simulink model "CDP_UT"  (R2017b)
settings: Solver=FixedStepDiscrete  StartTime=0.0  StopTime=10.0  FixedStep=0.01  RelTol=1e-3  EnableMultiTasking=on
undefined symbols (not defined in the file): ASWTYPE_FALSE, ASWTYPE_TRUE, CaCDP_CellTempNTCVoltTable_mV, CaCDP_CellTempTable_C, CaCDP_CMUPCBTempNTCVoltTable_mV, CaCDP_CMUPCBTempTable_C, CbCDP_DiffBusbarTempStateCheck_flg, CbCDP_DiffCellTempStateCheck_flg, CbCDP_DiffCellVoltStateCheck_flg, CbCDP_IgnorUpdateVld_flg, CbCDP_MaxBusbarTempStateCheck_flg, CbCDP_MaxCellTempStateCheck_flg, CbCDP_MaxCellVoltStateCheck_flg, CbCDP_MinBusbarTempStateCheck_flg, CbCDP_MinCellTempStateCheck_flg, CbCDP_MinCellVoltStateCheck_flg, CcCDP_AFETempConfig_numb, CcCDP_AFETempFltThd_C, CcCDP_AFETempFltThdHys_C, CcCDP_BusbarTempRngFltHiThrd_C, CcCDP_BusbarTempRngFltLowThrd_C, CcCDP_CellDiffFltLevel1_mV, CcCDP_CellDiffFltLevel2_mV, CcCDP_CellDiffFltLevel3_mV, CcCDP_CellTempLowerLimit_C, CcCDP_CellTempRngFltHiThrd_C, CcCDP_CellTempRngFltLowThrd_C, CcCDP_CellTempUpperLimit_C, CcCDP_CellVoltConfig_numb, CcCDP_CellVoltLowerLimit_mV, CcCDP_CellVoltRngHiThrd_mV, CcCDP_CellVoltRngLowThrd_mV, CcCDP_CellVoltUpdateThrd_numb, CcCDP_CellVoltUpperLimit_mV, CcCDP_ChrgMaxCellTempFltLv1Thrd_C, CcCDP_ChrgMaxCellTempFltLv2Thrd_C, CcCDP_ChrgMaxCellTempFltLv3Thrd_C, CcCDP_ChrgMaxCellTempReturnDiff_C, CcCDP_ChrgMinCellTempFltLv1Thrd_C, CcCDP_ChrgMinCellTempFltLv2Thrd_C, CcCDP_ChrgMinCellTempFltLv3Thrd_C, CcCDP_ChrgMinCellTempReturnDiff_C, CcCDP_CMUPCBTempConfig_numb, CcCDP_CMUPCBTempFltThd_C, CcCDP_CMUPCBTempFltThdHys_C, CcCDP_DiffBusbarTempFltLevel1Thrd_C, CcCDP_DiffBusbarTempFltLevel2Thrd_C, CcCDP_DiffBusbarTempReturnDifference_C, CcCDP_DiffCellTempFltLevel1Thrd_C, CcCDP_DiffCellTempFltLevel2Thrd_C, CcCDP_DiffCellTempReturnDifference_C, CcCDP_DiffCellVoltReturnDifference_mV, CcCDP_DiffVoltCheckMaxCellTempCondition_C, CcCDP_DiffVoltCheckMaxCellVoltCondition_mV, CcCDP_DiffVoltCheckMinCellTempCondition_C, CcCDP_DiffVoltCheckMinCellVoltCondition_mV, CcCDP_DiffVoltCheckPackCurrCondition_A, CcCDP_MaxAFETempIniVal_C, CcCDP_MaxBusbarTempFltLevel1Thrd_C, CcCDP_MaxBusbarTempFltLevel2Thrd_C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
libraries: AIWAYS_Powertrain_BMS_lib x148, simulink x8
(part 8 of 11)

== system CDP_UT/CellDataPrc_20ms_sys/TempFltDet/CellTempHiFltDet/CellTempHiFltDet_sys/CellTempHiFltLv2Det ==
  LbCDP_MaxTempCheckCondition_flg : Inport
  GcCDP_MaxCellTemp_C : Inport  Port=2
  Add1 : Sum  OutDataTypeStr=Inherit: Inherit via back propagation
  Add4 : Sum  OutDataTypeStr=Inherit: Inherit via back propagation
  CDP_GbCDP_ChrgMaxCellVoltFltLv1_flg : AIWAYS_Powertrain_BMS_lib/Signals/OverWrite  OverWrite_Value=CbCDP_CellTempHiFltLv2Ovr_flg  OverWrite_flag=CbCDP_CellTempHiFltLv2OvrSwt_flg
  Comparison : RelationalOperator  Operator=>  OutDataTypeStr=boolean
  Constant : Constant  Value=CcCDP_MaxCellTempFltLevel2Thrd_C
  Constant1 : Constant  Value=ASWTYPE_TRUE
  Constant2 : Constant  Value=CcCDP_MaxCellTempReturnDifference_C
  Constant3 : Constant  Value=CcCDP_MaxCellTempFltLevel3Thrd_C
  Constant4 : Constant  Value=CcCDP_MaxCellTempReturnDifference_C
  Constant5 : Constant  Value=ASWTYPE_TRUE
  Logical Operator : Logic  AllPortsSameDT=off  OutDataTypeStr=boolean
  Logical Operator1 : Logic  AllPortsSameDT=off  OutDataTypeStr=boolean
  Relational Operator : RelationalOperator  OutDataTypeStr=boolean
  Relational Operator1 : RelationalOperator  Operator===  OutDataTypeStr=boolean
  Terminator : Terminator
  GbCDP_CellTempHiFltLv2_flg : Outport
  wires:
  Constant2/1 -> Add4/2
  Logical Operator/1 -> CDP_GbCDP_ChrgMaxCellVoltFltLv1_flg/1
  Constant/1 -> Add4/1
  Add4/1 -> Relational Operator/2
  GcCDP_MaxCellTemp_C/1 -> Relational Operator/1, Comparison/2
  CDP_GbCDP_ChrgMaxCellVoltFltLv1_flg/1 -> GbCDP_CellTempHiFltLv2_flg/1  "GbCDP_CellTempHiFltLv2_flg"
  Relational Operator1/1 -> Logical Operator/2
  LbCDP_MaxTempCheckCondition_flg/1 -> Relational Operator1/1
  Constant1/1 -> Relational Operator1/2
  Relational Operator/1 -> Logical Operator1/2
  Constant4/1 -> Add1/2
  Constant3/1 -> Add1/1
  Add1/1 -> Comparison/1
  Comparison/1 -> Terminator/1
  Logical Operator1/1 -> Logical Operator/1
  Constant5/1 -> Logical Operator1/1

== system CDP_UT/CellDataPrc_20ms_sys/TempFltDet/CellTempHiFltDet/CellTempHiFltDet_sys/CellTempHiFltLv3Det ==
  LbCDP_MaxTempCheckCondition_flg : Inport
  GcCDP_MaxCellTemp_C : Inport  Port=2
  Add4 : Sum  OutDataTypeStr=Inherit: Inherit via back propagation
  CDP_GbCDP_ChrgMaxCellVoltFltLv1_flg : AIWAYS_Powertrain_BMS_lib/Signals/OverWrite  OverWrite_Value=CbCDP_CellTempHiFltLv3Ovr_flg  OverWrite_flag=CbCDP_CellTempHiFltLv3OvrSwt_flg
  Comparison : RelationalOperator  Operator=>  OutDataTypeStr=boolean
  Constant : Constant  Value=CcCDP_MaxCellTempFltLevel3Thrd_C
  Constant1 : Constant  Value=ASWTYPE_TRUE
  Constant2 : Constant  Value=CcCDP_MaxCellTempReturnDifference_C
  Constant3 : Constant  Value=CcCDP_CellTempRngFltHiThrd_C
  Constant4 : Constant  Value=ASWTYPE_TRUE
  Logical Operator : Logic  AllPortsSameDT=off  OutDataTypeStr=boolean
  Logical Operator1 : Logic  AllPortsSameDT=off  OutDataTypeStr=boolean
  Relational Operator : RelationalOperator  OutDataTypeStr=boolean
  Relational Operator1 : RelationalOperator  Operator===  OutDataTypeStr=boolean
  Terminator : Terminator
  GbCDP_CellTempHiFltLv3_flg : Outport
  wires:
  Logical Operator/1 -> CDP_GbCDP_ChrgMaxCellVoltFltLv1_flg/1
  CDP_GbCDP_ChrgMaxCellVoltFltLv1_flg/1 -> GbCDP_CellTempHiFltLv3_flg/1  "GbCDP_CellTempHiFltLv3_flg"
  Logical Operator1/1 -> Logical Operator/1
  Comparison/1 -> Terminator/1
  Relational Operator/1 -> Logical Operator1/2
  Constant/1 -> Add4/1
  Relational Operator1/1 -> Logical Operator/2
  Constant2/1 -> Add4/2
  Add4/1 -> Relational Operator/2
  LbCDP_MaxTempCheckCondition_flg/1 -> Relational Operator1/1
  Constant1/1 -> Relational Operator1/2
  GcCDP_MaxCellTemp_C/1 -> Relational Operator/1, Comparison/2
  Constant3/1 -> Comparison/1
  Constant4/1 -> Logical Operator1/1

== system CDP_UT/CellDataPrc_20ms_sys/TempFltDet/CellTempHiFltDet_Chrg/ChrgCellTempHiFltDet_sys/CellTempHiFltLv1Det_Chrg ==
  LbCDP_ChrgMaxTempChkCond_flg : Inport
  GcCDP_MaxCellTemp_C : Inport  Port=2
  Add1 : Sum  OutDataTypeStr=Inherit: Inherit via back propagation
  Add4 : Sum  OutDataTypeStr=Inherit: Inherit via back propagation
  CDP_GbCDP_ChrgMaxCellVoltFltLv1_flg : AIWAYS_Powertrain_BMS_lib/Signals/OverWrite  OverWrite_Value=CbCDP_ChrgCellTempHiFltLv1Ovr_flg  OverWrite_flag=CbCDP_ChrgCellTempHiFltLv1OvrSwt_flg
  Comparison : RelationalOperator  Operator=>  OutDataTypeStr=boolean
  Constant : Constant  Value=CcCDP_ChrgMaxCellTempFltLv1Thrd_C
  Constant1 : Constant  Value=ASWTYPE_TRUE
  Constant2 : Constant  Value=CcCDP_ChrgMaxCellTempReturnDiff_C
  Constant3 : Constant  Value=CcCDP_MaxCellTempFltLevel2Thrd_C
  Constant4 : Constant  Value=CcCDP_MaxCellTempReturnDifference_C
  Constant5 : Constant  Value=ASWTYPE_TRUE
  Logical Operator : Logic  AllPortsSameDT=off  OutDataTypeStr=boolean
  Logical Operator1 : Logic  AllPortsSameDT=off  OutDataTypeStr=boolean
  Relational Operator : RelationalOperator  OutDataTypeStr=boolean
  Relational Operator1 : RelationalOperator  Operator===  OutDataTypeStr=boolean
  Terminator : Terminator
  GbCDP_ChrgCellTempHiFltLv1_flg : Outport
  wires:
  Constant5/1 -> Logical Operator1/1
  GcCDP_MaxCellTemp_C/1 -> Comparison/2, Relational Operator/1
  Constant1/1 -> Relational Operator1/2
  LbCDP_ChrgMaxTempChkCond_flg/1 -> Relational Operator1/1
  Constant4/1 -> Add1/2
  Add4/1 -> Relational Operator/2
  Constant2/1 -> Add4/2
  Relational Operator1/1 -> Logical Operator/2
  Constant/1 -> Add4/1
  Relational Operator/1 -> Logical Operator1/2
  Constant3/1 -> Add1/1
  Comparison/1 -> Terminator/1
  Add1/1 -> Comparison/1
  Logical Operator1/1 -> Logical Operator/1
  CDP_GbCDP_ChrgMaxCellVoltFltLv1_flg/1 -> GbCDP_ChrgCellTempHiFltLv1_flg/1  "GbCDP_ChrgCellTempHiFltLv1_flg"
  Logical Operator/1 -> CDP_GbCDP_ChrgMaxCellVoltFltLv1_flg/1

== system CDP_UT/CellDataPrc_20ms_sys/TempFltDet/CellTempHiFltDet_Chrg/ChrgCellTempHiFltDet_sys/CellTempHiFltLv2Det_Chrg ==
  LbCDP_ChrgMaxTempChkCond_flg : Inport
  GcCDP_MaxCellTemp_C : Inport  Port=2
  Add1 : Sum  OutDataTypeStr=Inherit: Inherit via back propagation
  Add4 : Sum  OutDataTypeStr=Inherit: Inherit via back propagation
  CDP_GbCDP_ChrgMaxCellVoltFltLv1_flg : AIWAYS_Powertrain_BMS_lib/Signals/OverWrite  OverWrite_Value=CbCDP_ChrgCellTempHiFltLv2Ovr_flg  OverWrite_flag=CbCDP_ChrgCellTempHiFltLv2OvrSwt_flg
  Comparison : RelationalOperator  Operator=>  OutDataTypeStr=boolean
  Constant : Constant  Value=CcCDP_ChrgMaxCellTempFltLv2Thrd_C
  Constant1 : Constant  Value=ASWTYPE_TRUE
  Constant2 : Constant  Value=CcCDP_ChrgMaxCellTempReturnDiff_C
  Constant3 : Constant  Value=CcCDP_MaxCellTempFltLevel3Thrd_C
  Constant4 : Constant  Value=CcCDP_MaxCellTempReturnDifference_C
  Constant5 : Constant  Value=ASWTYPE_TRUE
  Logical Operator : Logic  AllPortsSameDT=off  OutDataTypeStr=boolean
  Logical Operator1 : Logic  AllPortsSameDT=off  OutDataTypeStr=boolean
  Relational Operator : RelationalOperator  OutDataTypeStr=boolean
  Relational Operator1 : RelationalOperator  Operator===  OutDataTypeStr=boolean
  Terminator : Terminator
  GbCDP_ChrgCellTempHiFltLv2_flg : Outport
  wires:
  Constant5/1 -> Logical Operator1/1
  Logical Operator1/1 -> Logical Operator/1
  Comparison/1 -> Terminator/1
  Add1/1 -> Comparison/1
  Constant3/1 -> Add1/1
  Constant4/1 -> Add1/2
  Relational Operator/1 -> Logical Operator1/2
  Constant1/1 -> Relational Operator1/2
  LbCDP_ChrgMaxTempChkCond_flg/1 -> Relational Operator1/1
  Relational Operator1/1 -> Logical Operator/2
  CDP_GbCDP_ChrgMaxCellVoltFltLv1_flg/1 -> GbCDP_ChrgCellTempHiFltLv2_flg/1  "GbCDP_ChrgCellTempHiFltLv2_flg"
  GcCDP_MaxCellTemp_C/1 -> Comparison/2, Relational Operator/1
  Add4/1 -> Relational Operator/2
  Constant/1 -> Add4/1
  Logical Operator/1 -> CDP_GbCDP_ChrgMaxCellVoltFltLv1_flg/1
  Constant2/1 -> Add4/2

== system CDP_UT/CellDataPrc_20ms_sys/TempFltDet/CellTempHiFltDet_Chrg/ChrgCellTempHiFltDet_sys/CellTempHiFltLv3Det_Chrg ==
  LbCDP_ChrgMaxTempChkCond_flg : Inport
  GcCDP_MaxCellTemp_C : Inport  Port=2
  Add4 : Sum  OutDataTypeStr=Inherit: Inherit via back propagation
  CDP_GbCDP_ChrgMaxCellVoltFltLv1_flg : AIWAYS_Powertrain_BMS_lib/Signals/OverWrite  OverWrite_Value=CbCDP_ChrgCellTempHiFltLv3Ovr_flg  OverWrite_flag=CbCDP_ChrgCellTempHiFltLv3OvrSwt_flg
  Comparison : RelationalOperator  Operator=>  OutDataTypeStr=boolean
  Constant : Constant  Value=CcCDP_ChrgMaxCellTempFltLv3Thrd_C
  Constant1 : Constant  Value=ASWTYPE_TRUE
  Constant2 : Constant  Value=CcCDP_ChrgMaxCellTempReturnDiff_C
  Constant3 : Constant  Value=CcCDP_CellTempRngFltHiThrd_C
  Constant4 : Constant  Value=ASWTYPE_TRUE
  Logical Operator : Logic  AllPortsSameDT=off  OutDataTypeStr=boolean
  Logical Operator1 : Logic  AllPortsSameDT=off  OutDataTypeStr=boolean
  Relational Operator : RelationalOperator  OutDataTypeStr=boolean
  Relational Operator1 : RelationalOperator  Operator===  OutDataTypeStr=boolean
  Terminator : Terminator
  GbCDP_ChrgCellTempHiFltLv3_flg : Outport
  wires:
  Constant4/1 -> Logical Operator1/1
  Constant3/1 -> Comparison/1
  GcCDP_MaxCellTemp_C/1 -> Comparison/2, Relational Operator/1
  Constant1/1 -> Relational Operator1/2
  LbCDP_ChrgMaxTempChkCond_flg/1 -> Relational Operator1/1
  Add4/1 -> Relational Operator/2
  Constant2/1 -> Add4/2
  Relational Operator1/1 -> Logical Operator/2
  Constant/1 -> Add4/1
  Relational Operator/1 -> Logical Operator1/2
  Comparison/1 -> Terminator/1
  Logical Operator1/1 -> Logical Operator/1
  CDP_GbCDP_ChrgMaxCellVoltFltLv1_flg/1 -> GbCDP_ChrgCellTempHiFltLv3_flg/1  "GbCDP_ChrgCellTempHiFltLv3_flg"
  Logical Operator/1 -> CDP_GbCDP_ChrgMaxCellVoltFltLv1_flg/1

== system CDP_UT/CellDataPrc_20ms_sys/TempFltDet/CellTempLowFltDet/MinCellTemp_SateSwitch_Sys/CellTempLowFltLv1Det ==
  GcCDP_MinCellTemp_C : Inport
  LbCDP_MinTempCheckCondition_flg : Inport  Port=2
  Add1 : Sum  Inputs=+-  OutDataTypeStr=Inherit: Inherit via back propagation
  Add4 : Sum  Inputs=+-  OutDataTypeStr=Inherit: Inherit via back propagation
  CDP_GbCDP_ChrgMaxCellVoltFltLv1_flg : AIWAYS_Powertrain_BMS_lib/Signals/OverWrite  OverWrite_Value=CbCDP_CellTempLowFltLv1Ovr_flg  OverWrite_flag=CbCDP_CellTempLowFltLv1OvrSwt_flg
  Comparison2 : RelationalOperator  Operator=<  OutDataTypeStr=boolean
  Constant : Constant  Value=CcCDP_MinCellTempFltLevel1Thrd_C
  Constant1 : Constant  Value=ASWTYPE_TRUE
  Constant2 : Constant  Value=CcCDP_MinCellTempReturnDifference_C
  Constant3 : Constant  Value=CcCDP_MinCellTempFltLevel2Thrd_C
  Constant4 : Constant  Value=CcCDP_MinCellTempReturnDifference_C
  Constant5 : Constant  Value=ASWTYPE_TRUE
  Logical Operator : Logic  AllPortsSameDT=off  OutDataTypeStr=boolean
  Logical Operator1 : Logic  AllPortsSameDT=off  OutDataTypeStr=boolean
  Relational Operator : RelationalOperator  Operator=<=  OutDataTypeStr=boolean
  Relational Operator1 : RelationalOperator  Operator===  OutDataTypeStr=boolean
  Terminator : Terminator
  GbCDP_CellTempLowFltLv1_flg : Outport
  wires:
  Logical Operator/1 -> CDP_GbCDP_ChrgMaxCellVoltFltLv1_flg/1
  CDP_GbCDP_ChrgMaxCellVoltFltLv1_flg/1 -> GbCDP_CellTempLowFltLv1_flg/1  "GbCDP_CellTempLowFltLv1_flg"
  Constant1/1 -> Relational Operator1/2
  LbCDP_MinTempCheckCondition_flg/1 -> Relational Operator1/1
  Constant2/1 -> Add4/2
  Add4/1 -> Relational Operator/2
  Relational Operator1/1 -> Logical Operator/2
  Add1/1 -> Comparison2/1
  Comparison2/1 -> Terminator/1
  Logical Operator1/1 -> Logical Operator/1
  Relational Operator/1 -> Logical Operator1/2
  Constant/1 -> Add4/1
  Constant4/1 -> Add1/2
  GcCDP_MinCellTemp_C/1 -> Relational Operator/1, Comparison2/2
  Constant3/1 -> Add1/1
  Constant5/1 -> Logical Operator1/1

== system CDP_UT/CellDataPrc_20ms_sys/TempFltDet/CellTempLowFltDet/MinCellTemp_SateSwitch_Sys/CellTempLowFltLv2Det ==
  GcCDP_MinCellTemp_C : Inport
  LbCDP_MinTempCheckCondition_flg : Inport  Port=2
  Add1 : Sum  Inputs=+-  OutDataTypeStr=Inherit: Inherit via back propagation
  Add4 : Sum  Inputs=+-  OutDataTypeStr=Inherit: Inherit via back propagation
  CDP_GbCDP_ChrgMaxCellVoltFltLv1_flg : AIWAYS_Powertrain_BMS_lib/Signals/OverWrite  OverWrite_Value=CbCDP_CellTempLowFltLv2Ovr_flg  OverWrite_flag=CbCDP_CellTempLowFltLv2OvrSwt_flg
  Comparison2 : RelationalOperator  Operator=<  OutDataTypeStr=boolean
  Constant : Constant  Value=CcCDP_MinCellTempFltLevel2Thrd_C
  Constant1 : Constant  Value=ASWTYPE_TRUE
  Constant2 : Constant  Value=CcCDP_MinCellTempReturnDifference_C
  Constant3 : Constant  Value=CcCDP_MinCellTempFltLevel3Thrd_C
  Constant4 : Constant  Value=CcCDP_MinCellTempReturnDifference_C
  Constant5 : Constant  Value=ASWTYPE_TRUE
  Logical Operator : Logic  AllPortsSameDT=off  OutDataTypeStr=boolean
  Logical Operator1 : Logic  AllPortsSameDT=off  OutDataTypeStr=boolean
  Relational Operator : RelationalOperator  Operator=<=  OutDataTypeStr=boolean
  Relational Operator1 : RelationalOperator  Operator===  OutDataTypeStr=boolean
  Terminator : Terminator
  GbCDP_CellTempLowFltLv2_flg : Outport
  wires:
  Constant/1 -> Add4/1
  GcCDP_MinCellTemp_C/1 -> Relational Operator/1, Comparison2/2
  Constant2/1 -> Add4/2
  Add4/1 -> Relational Operator/2
  Logical Operator/1 -> CDP_GbCDP_ChrgMaxCellVoltFltLv1_flg/1
  LbCDP_MinTempCheckCondition_flg/1 -> Relational Operator1/1
  Relational Operator1/1 -> Logical Operator/2
  Constant1/1 -> Relational Operator1/2
  CDP_GbCDP_ChrgMaxCellVoltFltLv1_flg/1 -> GbCDP_CellTempLowFltLv2_flg/1  "GbCDP_CellTempLowFltLv2_flg"
  Relational Operator/1 -> Logical Operator1/2
  Constant4/1 -> Add1/2
  Constant3/1 -> Add1/1
  Add1/1 -> Comparison2/1
  Comparison2/1 -> Terminator/1
  Logical Operator1/1 -> Logical Operator/1
  Constant5/1 -> Logical Operator1/1

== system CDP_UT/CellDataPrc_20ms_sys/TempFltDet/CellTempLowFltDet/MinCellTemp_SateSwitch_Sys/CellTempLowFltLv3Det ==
  GcCDP_MinCellTemp_C : Inport
  LbCDP_MinTempCheckCondition_flg : Inport  Port=2
  Add4 : Sum  Inputs=+-  OutDataTypeStr=Inherit: Inherit via back propagation
  CDP_GbCDP_ChrgMaxCellVoltFltLv1_flg : AIWAYS_Powertrain_BMS_lib/Signals/OverWrite  OverWrite_Value=CbCDP_CellTempLowFltLv3Ovr_flg  OverWrite_flag=CbCDP_CellTempLowFltLv3OvrSwt_flg
  Comparison2 : RelationalOperator  Operator=<  OutDataTypeStr=boolean
  Constant : Constant  Value=CcCDP_MinCellTempFltLevel3Thrd_C
  Constant1 : Constant  Value=ASWTYPE_TRUE
  Constant2 : Constant  Value=CcCDP_MinCellTempReturnDifference_C
  Constant3 : Constant  Value=CcCDP_CellTempRngFltHiThrd_C
  Constant4 : Constant  Value=ASWTYPE_TRUE
  Logical Operator : Logic  AllPortsSameDT=off  OutDataTypeStr=boolean
  Logical Operator1 : Logic  AllPortsSameDT=off  OutDataTypeStr=boolean
  Relational Operator : RelationalOperator  Operator=<=  OutDataTypeStr=boolean
  Relational Operator1 : RelationalOperator  Operator===  OutDataTypeStr=boolean
  Terminator : Terminator
  GbCDP_CellTempLowFltLv3_flg : Outport
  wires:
  Logical Operator/1 -> CDP_GbCDP_ChrgMaxCellVoltFltLv1_flg/1
  CDP_GbCDP_ChrgMaxCellVoltFltLv1_flg/1 -> GbCDP_CellTempLowFltLv3_flg/1  "GbCDP_CellTempLowFltLv3_flg"
  Constant1/1 -> Relational Operator1/2
  LbCDP_MinTempCheckCondition_flg/1 -> Relational Operator1/1
  Constant2/1 -> Add4/2
  Add4/1 -> Relational Operator/2
  Relational Operator1/1 -> Logical Operator/2
  Comparison2/1 -> Terminator/1
  Logical Operator1/1 -> Logical Operator/1
  Relational Operator/1 -> Logical Operator1/2
  Constant/1 -> Add4/1
  GcCDP_MinCellTemp_C/1 -> Comparison2/2, Relational Operator/1
  Constant3/1 -> Comparison2/1
  Constant4/1 -> Logical Operator1/1

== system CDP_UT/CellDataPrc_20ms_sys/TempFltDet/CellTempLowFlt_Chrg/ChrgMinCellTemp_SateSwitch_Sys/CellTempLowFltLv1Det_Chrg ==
  GcCDP_MinCellTemp_C : Inport
  LbCDP_ChrgMinTempChkCond_flg : Inport  Port=2
  Add1 : Sum  Inputs=+-  OutDataTypeStr=Inherit: Inherit via back propagation
  Add4 : Sum  Inputs=+-  OutDataTypeStr=Inherit: Inherit via back propagation
  CDP_GbCDP_ChrgMaxCellVoltFltLv1_flg : AIWAYS_Powertrain_BMS_lib/Signals/OverWrite  OverWrite_Value=CbCDP_ChrgCellTempLowFltLv1Ovr_flg  OverWrite_flag=CbCDP_ChrgCellTempLowFltLv1OvrSwt_flg
  Comparison2 : RelationalOperator  Operator=<  OutDataTypeStr=boolean
  Constant : Constant  Value=CcCDP_ChrgMinCellTempFltLv1Thrd_C
  Constant1 : Constant  Value=ASWTYPE_TRUE
  Constant2 : Constant  Value=CcCDP_ChrgMinCellTempReturnDiff_C
  Constant3 : Constant  Value=CcCDP_MinCellTempFltLevel2Thrd_C
  Constant4 : Constant  Value=CcCDP_MinCellTempReturnDifference_C
  Constant5 : Constant  Value=ASWTYPE_TRUE
  Logical Operator : Logic  AllPortsSameDT=off  OutDataTypeStr=boolean
  Logical Operator1 : Logic  AllPortsSameDT=off  OutDataTypeStr=boolean
  Relational Operator : RelationalOperator  Operator=<=  OutDataTypeStr=boolean
  Relational Operator1 : RelationalOperator  Operator===  OutDataTypeStr=boolean
  Terminator : Terminator
  GbCDP_ChrgCellTempLowFltLv1_flg : Outport
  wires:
  Constant5/1 -> Logical Operator1/1
  Constant3/1 -> Add1/1
  GcCDP_MinCellTemp_C/1 -> Comparison2/2, Relational Operator/1
  Constant4/1 -> Add1/2
  Constant/1 -> Add4/1
  Relational Operator/1 -> Logical Operator1/2
  Logical Operator1/1 -> Logical Operator/1
  Comparison2/1 -> Terminator/1
  Add1/1 -> Comparison2/1
  Relational Operator1/1 -> Logical Operator/2
  Add4/1 -> Relational Operator/2
  Constant2/1 -> Add4/2
  LbCDP_ChrgMinTempChkCond_flg/1 -> Relational Operator1/1
  Constant1/1 -> Relational Operator1/2
  CDP_GbCDP_ChrgMaxCellVoltFltLv1_flg/1 -> GbCDP_ChrgCellTempLowFltLv1_flg/1  "GbCDP_ChrgCellTempLowFltLv1_flg"
  Logical Operator/1 -> CDP_GbCDP_ChrgMaxCellVoltFltLv1_flg/1

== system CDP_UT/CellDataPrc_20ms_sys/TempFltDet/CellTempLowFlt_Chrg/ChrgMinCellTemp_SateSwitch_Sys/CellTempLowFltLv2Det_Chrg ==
  GcCDP_MinCellTemp_C : Inport
  LbCDP_ChrgMinTempChkCond_flg : Inport  Port=2
  Add1 : Sum  Inputs=+-  OutDataTypeStr=Inherit: Inherit via back propagation
  Add4 : Sum  Inputs=+-  OutDataTypeStr=Inherit: Inherit via back propagation
  CDP_GbCDP_ChrgMaxCellVoltFltLv1_flg : AIWAYS_Powertrain_BMS_lib/Signals/OverWrite  OverWrite_Value=CbCDP_ChrgCellTempLowFltLv2Ovr_flg  OverWrite_flag=CbCDP_ChrgCellTempLowFltLv2OvrSwt_flg
  Comparison2 : RelationalOperator  Operator=<  OutDataTypeStr=boolean
  Constant : Constant  Value=CcCDP_ChrgMinCellTempFltLv2Thrd_C
  Constant1 : Constant  Value=ASWTYPE_TRUE
  Constant2 : Constant  Value=CcCDP_ChrgMinCellTempReturnDiff_C
  Constant3 : Constant  Value=CcCDP_MinCellTempFltLevel3Thrd_C
  Constant4 : Constant  Value=CcCDP_MinCellTempReturnDifference_C
  Constant5 : Constant  Value=ASWTYPE_TRUE
  Logical Operator : Logic  AllPortsSameDT=off  OutDataTypeStr=boolean
  Logical Operator1 : Logic  AllPortsSameDT=off  OutDataTypeStr=boolean
  Relational Operator : RelationalOperator  Operator=<=  OutDataTypeStr=boolean
  Relational Operator1 : RelationalOperator  Operator===  OutDataTypeStr=boolean
  Terminator : Terminator
  GbCDP_ChrgCellTempLowFltLv2_flg : Outport
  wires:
  Constant5/1 -> Logical Operator1/1
  Logical Operator1/1 -> Logical Operator/1
  Comparison2/1 -> Terminator/1
  Add1/1 -> Comparison2/1
  Constant3/1 -> Add1/1
  Constant4/1 -> Add1/2
  Relational Operator/1 -> Logical Operator1/2
  CDP_GbCDP_ChrgMaxCellVoltFltLv1_flg/1 -> GbCDP_ChrgCellTempLowFltLv2_flg/1  "GbCDP_ChrgCellTempLowFltLv2_flg"
  Constant1/1 -> Relational Operator1/2
  Relational Operator1/1 -> Logical Operator/2
  LbCDP_ChrgMinTempChkCond_flg/1 -> Relational Operator1/1
  Logical Operator/1 -> CDP_GbCDP_ChrgMaxCellVoltFltLv1_flg/1
  Add4/1 -> Relational Operator/2
  Constant2/1 -> Add4/2
  GcCDP_MinCellTemp_C/1 -> Comparison2/2, Relational Operator/1
  Constant/1 -> Add4/1

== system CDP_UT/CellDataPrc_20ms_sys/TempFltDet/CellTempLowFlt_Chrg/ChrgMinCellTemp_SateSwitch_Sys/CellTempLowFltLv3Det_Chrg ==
  GcCDP_MinCellTemp_C : Inport
  LbCDP_ChrgMinTempChkCond_flg : Inport  Port=2
  Add4 : Sum  Inputs=+-  OutDataTypeStr=Inherit: Inherit via back propagation
  CDP_GbCDP_ChrgMaxCellVoltFltLv1_flg : AIWAYS_Powertrain_BMS_lib/Signals/OverWrite  OverWrite_Value=CbCDP_ChrgCellTempLowFltLv3Ovr_flg  OverWrite_flag=CbCDP_ChrgCellTempLowFltLv3OvrSwt_flg
  Comparison2 : RelationalOperator  Operator=<  OutDataTypeStr=boolean
  Constant : Constant  Value=CcCDP_ChrgMinCellTempFltLv3Thrd_C
  Constant1 : Constant  Value=ASWTYPE_TRUE
  Constant2 : Constant  Value=CcCDP_ChrgMinCellTempReturnDiff_C
  Constant3 : Constant  Value=CcCDP_CellTempRngFltHiThrd_C
  Constant4 : Constant  Value=ASWTYPE_TRUE
  Logical Operator : Logic  AllPortsSameDT=off  OutDataTypeStr=boolean
  Logical Operator1 : Logic  AllPortsSameDT=off  OutDataTypeStr=boolean
  Relational Operator : RelationalOperator  Operator=<=  OutDataTypeStr=boolean
  Relational Operator1 : RelationalOperator  Operator===  OutDataTypeStr=boolean
  Terminator : Terminator
  GbCDP_ChrgCellTempLowFltLv3_flg : Outport
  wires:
  Constant4/1 -> Logical Operator1/1
  Constant3/1 -> Comparison2/1
  GcCDP_MinCellTemp_C/1 -> Relational Operator/1, Comparison2/2
  Constant/1 -> Add4/1
  Relational Operator/1 -> Logical Operator1/2
  Logical Operator1/1 -> Logical Operator/1
  Comparison2/1 -> Terminator/1
  Relational Operator1/1 -> Logical Operator/2
  Add4/1 -> Relational Operator/2
  Constant2/1 -> Add4/2
  LbCDP_ChrgMinTempChkCond_flg/1 -> Relational Operator1/1
  Constant1/1 -> Relational Operator1/2
  CDP_GbCDP_ChrgMaxCellVoltFltLv1_flg/1 -> GbCDP_ChrgCellTempLowFltLv3_flg/1  "GbCDP_ChrgCellTempLowFltLv3_flg"
  Logical Operator/1 -> CDP_GbCDP_ChrgMaxCellVoltFltLv1_flg/1

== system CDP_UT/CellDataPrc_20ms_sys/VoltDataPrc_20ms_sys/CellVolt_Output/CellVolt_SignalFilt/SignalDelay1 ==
  u : Inport
  Bus to Vector : BusToVector
  Delay1Cycle : Subsystem
  Delay2Cycle : Subsystem
  Delay3Cycle : Subsystem
  Delay4Cycle : Subsystem
  Mux : Mux  Inputs=5
  y : Outport
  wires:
  u/1 -> Mux/1, Delay4Cycle/1(u), Delay3Cycle/1(u), Delay2Cycle/1(u), Delay1Cycle/1(u)
  Bus to Vector/1 -> y/1
  Delay4Cycle/1(y) -> Mux/5
  Delay2Cycle/1(y) -> Mux/3
  Delay3Cycle/1(y) -> Mux/4
  Delay1Cycle/1(y) -> Mux/2
  Mux/1 -> Bus to Vector/1

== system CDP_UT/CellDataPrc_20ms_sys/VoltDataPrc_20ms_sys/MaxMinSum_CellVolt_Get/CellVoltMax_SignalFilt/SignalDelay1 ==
  u : Inport
  Bus to Vector : BusToVector
  Delay1Cycle : Subsystem
  Delay2Cycle : Subsystem
  Delay3Cycle : Subsystem
  Delay4Cycle : Subsystem
  Mux : Mux  Inputs=5
  y : Outport
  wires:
  u/1 -> Mux/1, Delay4Cycle/1(u), Delay3Cycle/1(u), Delay2Cycle/1(u), Delay1Cycle/1(u)
  Bus to Vector/1 -> y/1
  Delay4Cycle/1(y) -> Mux/5
  Delay2Cycle/1(y) -> Mux/3
  Delay3Cycle/1(y) -> Mux/4
  Delay1Cycle/1(y) -> Mux/2
  Mux/1 -> Bus to Vector/1

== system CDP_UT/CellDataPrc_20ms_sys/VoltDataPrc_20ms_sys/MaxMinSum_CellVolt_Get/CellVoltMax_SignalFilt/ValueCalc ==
  Output_Value : Inport
  Output_index : Inport  Port=2
  CcCDP_CellVoltFilConfig_numb : Inport  Port=3
  Constant2 : Constant  Value=CDP_CONST1_NUMB
  Constant4 : Constant  Value=CDP_CONST2_NUMB
  Constant6 : Constant  Value=CDP_CONST1_NUMB
  Constant7 : Constant  Value=CDP_CONST2_NUMB
  Product1 : Product  Inputs=*/  OutDataTypeStr=Inherit: Inherit via back propagation
  Product2 : Product  Inputs=*/  OutDataTypeStr=Inherit: Inherit via back propagation
  Selector : Selector  InputPortWidth=5  IndexOptions=Index vector (port)  Indices=[1 3]  OutputSizes=1
  Selector1 : Selector  InputPortWidth=5  IndexOptions=Index vector (port)  Indices=[1 3]  OutputSizes=1
  Sum : Sum  OutDataTypeStr=Inherit: Inherit via back propagation  RndMeth=Zero
  Sum1 : Sum  OutDataTypeStr=Inherit: Inherit via back propagation  RndMeth=Zero
  GcCDP_MaxCellVolt_mV : Outport
  Output_index1 : Outport  Port=2
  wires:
  Selector1/1 -> Output_index1/1
  Selector/1 -> GcCDP_MaxCellVolt_mV/1
  Sum1/1 -> Product2/1
  Constant7/1 -> Product2/2
  Constant2/1 -> Sum/2
  Output_Value/1 -> Selector/1
  Constant6/1 -> Sum1/2
  Output_index/1 -> Selector1/1
  Sum/1 -> Product1/1
  Constant4/1 -> Product1/2
  Product1/1 -> Selector/2
  Product2/1 -> Selector1/2
  CcCDP_CellVoltFilConfig_numb/1 -> Sum/1, Sum1/1

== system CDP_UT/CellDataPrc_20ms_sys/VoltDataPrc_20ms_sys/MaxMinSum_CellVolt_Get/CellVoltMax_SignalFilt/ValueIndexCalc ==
  Output_index1 : Inport
  LcCDP_MaxCellVoltNumb_numb : Inport  Port=2
  LbCDP_CellVoltUpdateVld_flg : Inport  Port=3
  InputValueCalc1 : Stateflow chart  TreatAsAtomicUnit=on
  Selector2 : Selector  IndexMode=Zero-based  InputPortWidth=5  IndexOptions=Index vector (port)  Indices=[1 3]  OutputSizes=1
  Unit Delay1 : UnitDelay  SampleTime=-1  StateName=StateName
  GcCDP_MaxCellVoltNumb_numb : Outport
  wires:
  LbCDP_CellVoltUpdateVld_flg/1 -> InputValueCalc1/2(Rige)
  Output_index1/1 -> Selector2/2
  InputValueCalc1/1(Output_Value) -> Selector2/1, Unit Delay1/1
  Unit Delay1/1 -> InputValueCalc1/3(Old_Value)
  LcCDP_MaxCellVoltNumb_numb/1 -> InputValueCalc1/1(Input_Value)
  Selector2/1 -> GcCDP_MaxCellVoltNumb_numb/1

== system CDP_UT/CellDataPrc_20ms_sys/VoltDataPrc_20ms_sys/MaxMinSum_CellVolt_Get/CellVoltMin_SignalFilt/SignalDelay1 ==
  u : Inport
  Bus to Vector : BusToVector
  Delay1Cycle : Subsystem
  Delay2Cycle : Subsystem
  Delay3Cycle : Subsystem
  Delay4Cycle : Subsystem
  Mux : Mux  Inputs=5
  y : Outport
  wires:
  Mux/1 -> Bus to Vector/1
  Delay1Cycle/1(y) -> Mux/2
  Delay3Cycle/1(y) -> Mux/4
  Delay2Cycle/1(y) -> Mux/3
  Delay4Cycle/1(y) -> Mux/5
  Bus to Vector/1 -> y/1
  u/1 -> Delay1Cycle/1(u), Delay2Cycle/1(u), Delay3Cycle/1(u), Delay4Cycle/1(u), Mux/1

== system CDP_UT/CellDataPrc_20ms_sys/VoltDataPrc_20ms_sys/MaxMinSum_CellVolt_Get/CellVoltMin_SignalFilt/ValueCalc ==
  Output_Value : Inport
  Output_index : Inport  Port=2
  CcCDP_CellVoltFilConfig_numb : Inport  Port=3
  Constant2 : Constant  Value=CDP_CONST1_NUMB
  Constant4 : Constant  Value=CDP_CONST2_NUMB
  Constant6 : Constant  Value=CDP_CONST1_NUMB
  Constant7 : Constant  Value=CDP_CONST2_NUMB
  Product1 : Product  Inputs=*/  OutDataTypeStr=Inherit: Inherit via back propagation
  Product2 : Product  Inputs=*/  OutDataTypeStr=Inherit: Inherit via back propagation
  Selector : Selector  InputPortWidth=5  IndexOptions=Index vector (port)  Indices=[1 3]  OutputSizes=1
  Selector1 : Selector  InputPortWidth=5  IndexOptions=Index vector (port)  Indices=[1 3]  OutputSizes=1
  Sum : Sum  OutDataTypeStr=Inherit: Inherit via back propagation  RndMeth=Zero
  Sum1 : Sum  OutDataTypeStr=Inherit: Inherit via back propagation  RndMeth=Zero
  GcCDP_MinCellVolt_mV : Outport
  Output_index1 : Outport  Port=2
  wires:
  CcCDP_CellVoltFilConfig_numb/1 -> Sum1/1, Sum/1
  Product2/1 -> Selector1/2
  Product1/1 -> Selector/2
  Constant4/1 -> Product1/2
  Sum/1 -> Product1/1
  Output_index/1 -> Selector1/1
  Constant6/1 -> Sum1/2
  Output_Value/1 -> Selector/1
  Constant2/1 -> Sum/2
  Constant7/1 -> Product2/2
  Sum1/1 -> Product2/1
  Selector/1 -> GcCDP_MinCellVolt_mV/1
  Selector1/1 -> Output_index1/1

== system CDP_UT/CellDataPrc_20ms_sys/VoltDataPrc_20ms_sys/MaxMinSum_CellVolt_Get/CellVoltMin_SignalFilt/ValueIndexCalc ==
  Output_index1 : Inport
  LcCDP_MinCellVoltNumb_numb : Inport  Port=2
  LbCDP_CellVoltUpdateVld_flg : Inport  Port=3
  InputValueCalc1 : Stateflow chart  TreatAsAtomicUnit=on
  Selector2 : Selector  IndexMode=Zero-based  InputPortWidth=5  IndexOptions=Index vector (port)  Indices=[1 3]  OutputSizes=1
  Unit Delay1 : UnitDelay  SampleTime=-1  StateName=StateName
  GcCDP_MinCellVoltNumb_numb : Outport
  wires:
  LcCDP_MinCellVoltNumb_numb/1 -> InputValueCalc1/1(Input_Value)
  Unit Delay1/1 -> InputValueCalc1/3(Old_Value)
  InputValueCalc1/1(Output_Value) -> Unit Delay1/1, Selector2/1
  Output_index1/1 -> Selector2/2
  LbCDP_CellVoltUpdateVld_flg/1 -> InputValueCalc1/2(Rige)
  Selector2/1 -> GcCDP_MinCellVoltNumb_numb/1

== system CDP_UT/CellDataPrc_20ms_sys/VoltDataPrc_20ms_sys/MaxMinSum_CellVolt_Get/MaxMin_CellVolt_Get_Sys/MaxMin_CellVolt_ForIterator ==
  CcCDP_CellVoltConfig_numb : Inport
  LaCDP_CellVolt_mV : Inport  Port=2
  LaCDP_CellVoltVld_flg : Inport  Port=3
  Bus Creator : BusCreator  Inputs=3
  Bus Selector1 : BusSelector  OutputSignals=LcCDP_IniOutputCellVolt_mV,LcCDP_IniOutputCellVoltNumb_numb,LbCDP_IniOutputCellVoltVld_flg
  Bus Selector2 : BusSelector  OutputSignals=LcCDP_IniOutputCellVolt_mV,LcCDP_IniOutputCellVoltNumb_numb,LbCDP_IniOutputCellVoltVld_flg
  Data Type Conversion : DataTypeConversion
  MaxCellVoltNumbIterator : ForIterator  ResetStates=reset  IterationSource=external  IterationVariableDataType=int16
  MaxCellVoltNumb_ForIterator : Subsystem
  MinCellVoltNumb_ForIterator : Subsystem
  Selector : Selector  IndexOptions=Index vector (port)  Indices=[1 3]  OutputSizes=1
  Selector1 : Selector  IndexOptions=Index vector (port)  Indices=[1 3]  OutputSizes=1
  LcCDP_MaxCellVolt_mV : Outport
  LcCDP_MaxCellVoltNumb_numb : Outport  Port=2
  LcCDP_MinCellVolt_mV : Outport  Port=3
  LcCDP_MinCellVoltNumb_numb : Outport  Port=4
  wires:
  Bus Selector2/2 -> MinCellVoltNumb_ForIterator/2(LcCDP_IniOutputCellVoltNumb_numb)  "<LcCDP_IniOutputCellVoltNumb_numb>"
  Bus Selector2/1 -> MinCellVoltNumb_ForIterator/1(LcCDP_IniOutputCellVolt_mV)  "<LcCDP_IniOutputCellVolt_mV>"
  Bus Selector1/2 -> MaxCellVoltNumb_ForIterator/2(LcCDP_IniOutputCellVoltNumb_numb)  "<LcCDP_IniOutputCellVoltNumb_numb>"
  Bus Selector1/1 -> MaxCellVoltNumb_ForIterator/1(LcCDP_IniOutputCellVolt_mV)  "<LcCDP_IniOutputCellVolt_mV>"
  Data Type Conversion/1 -> Bus Creator/2  "LcCDP_IniOutputCellVoltNumb_numb"
  Bus Creator/1 -> Bus Selector2/1, Bus Selector1/1
  Selector/1 -> Bus Creator/1  "LcCDP_IniOutputCellVolt_mV"
  MaxCellVoltNumbIterator/1 -> Selector1/2, Data Type Conversion/1, Selector/2
  LaCDP_CellVolt_mV/1 -> Selector/1
  CcCDP_CellVoltConfig_numb/1 -> MaxCellVoltNumbIterator/1
  MaxCellVoltNumb_ForIterator/1(LcCDP_MaxCellVolt_mV) -> LcCDP_MaxCellVolt_mV/1
  MaxCellVoltNumb_ForIterator/2(LcCDP_MaxCellVoltNumb_numb) -> LcCDP_MaxCellVoltNumb_numb/1
  MinCellVoltNumb_ForIterator/1(LcCDP_MinCellVolt_mV) -> LcCDP_MinCellVolt_mV/1
  MinCellVoltNumb_ForIterator/2(LcCDP_MinCellVoltNumb_numb) -> LcCDP_MinCellVoltNumb_numb/1
  LaCDP_CellVoltVld_flg/1 -> Selector1/1
  Selector1/1 -> Bus Creator/3  "LbCDP_IniOutputCellVoltVld_flg"
  Bus Selector1/3 -> MaxCellVoltNumb_ForIterator/3(LbCDP_IniOutputCellVoltVld_flg)  "<LbCDP_IniOutputCellVoltVld_flg>"
  Bus Selector2/3 -> MinCellVoltNumb_ForIterator/3(LbCDP_IniOutputCellVoltVld_flg)  "<LbCDP_IniOutputCellVoltVld_flg>"

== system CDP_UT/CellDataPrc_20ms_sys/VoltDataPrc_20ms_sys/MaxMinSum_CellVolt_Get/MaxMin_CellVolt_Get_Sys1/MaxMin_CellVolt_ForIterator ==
  CcCDP_CellVoltConfig_numb : Inport
  LaCDP_CellVolt_mV : Inport  Port=2
  LaCDP_CellVoltVld_flg : Inport  Port=3
  Bus Creator : BusCreator  Inputs=3
  Bus Selector1 : BusSelector  OutputSignals=LcCDP_IniOutputCellVolt_mV,LcCDP_IniOutputCellVoltNumb_numb,LbCDP_IniOutputCellVoltVld_flg
  Bus Selector2 : BusSelector  OutputSignals=LcCDP_IniOutputCellVolt_mV,LcCDP_IniOutputCellVoltNumb_numb,LbCDP_IniOutputCellVoltVld_flg
  Data Type Conversion : DataTypeConversion
  MaxCellVoltNumbIterator : ForIterator  ResetStates=reset  IterationSource=external  IterationVariableDataType=int16
  MaxCellVoltNumb_ForIterator : Subsystem
  MinCellVoltNumb_ForIterator : Subsystem
  Selector : Selector  IndexOptions=Index vector (port)  Indices=[1 3]  OutputSizes=1
  Selector1 : Selector  IndexOptions=Index vector (port)  Indices=[1 3]  OutputSizes=1
  LcCDP_MaxCellVolt_mV : Outport
  LcCDP_MaxCellVoltNumb_numb : Outport  Port=2
  LcCDP_MinCellVolt_mV : Outport  Port=3
  LcCDP_MinCellVoltNumb_numb : Outport  Port=4
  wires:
  Bus Selector2/3 -> MinCellVoltNumb_ForIterator/3(LbCDP_IniOutputCellVoltVld_flg)  "<LbCDP_IniOutputCellVoltVld_flg>"
  Bus Selector1/3 -> MaxCellVoltNumb_ForIterator/3(LbCDP_IniOutputCellVoltVld_flg)  "<LbCDP_IniOutputCellVoltVld_flg>"
  Selector1/1 -> Bus Creator/3  "LbCDP_IniOutputCellVoltVld_flg"
  LaCDP_CellVoltVld_flg/1 -> Selector1/1
  MinCellVoltNumb_ForIterator/2(LcCDP_MinCellVoltNumb_numb) -> LcCDP_MinCellVoltNumb_numb/1
  MinCellVoltNumb_ForIterator/1(LcCDP_MinCellVolt_mV) -> LcCDP_MinCellVolt_mV/1
  MaxCellVoltNumb_ForIterator/2(LcCDP_MaxCellVoltNumb_numb) -> LcCDP_MaxCellVoltNumb_numb/1
  MaxCellVoltNumb_ForIterator/1(LcCDP_MaxCellVolt_mV) -> LcCDP_MaxCellVolt_mV/1
  CcCDP_CellVoltConfig_numb/1 -> MaxCellVoltNumbIterator/1
  LaCDP_CellVolt_mV/1 -> Selector/1
  MaxCellVoltNumbIterator/1 -> Selector/2, Data Type Conversion/1, Selector1/2
  Selector/1 -> Bus Creator/1  "LcCDP_IniOutputCellVolt_mV"
  Bus Creator/1 -> Bus Selector1/1, Bus Selector2/1
  Data Type Conversion/1 -> Bus Creator/2  "LcCDP_IniOutputCellVoltNumb_numb"
  Bus Selector1/1 -> MaxCellVoltNumb_ForIterator/1(LcCDP_IniOutputCellVolt_mV)  "<LcCDP_IniOutputCellVolt_mV>"
  Bus Selector1/2 -> MaxCellVoltNumb_ForIterator/2(LcCDP_IniOutputCellVoltNumb_numb)  "<LcCDP_IniOutputCellVoltNumb_numb>"
  Bus Selector2/1 -> MinCellVoltNumb_ForIterator/1(LcCDP_IniOutputCellVolt_mV)  "<LcCDP_IniOutputCellVolt_mV>"
  Bus Selector2/2 -> MinCellVoltNumb_ForIterator/2(LcCDP_IniOutputCellVoltNumb_numb)  "<LcCDP_IniOutputCellVoltNumb_numb>"

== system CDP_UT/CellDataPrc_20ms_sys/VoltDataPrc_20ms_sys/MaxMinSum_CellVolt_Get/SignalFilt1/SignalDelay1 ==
  u : Inport
  Bus to Vector : BusToVector
  Delay1Cycle : Subsystem
  Delay2Cycle : Subsystem
  Delay3Cycle : Subsystem
  Delay4Cycle : Subsystem
  Mux : Mux  Inputs=5
  y : Outport
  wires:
  Mux/1 -> Bus to Vector/1
  Delay1Cycle/1(y) -> Mux/2
  Delay3Cycle/1(y) -> Mux/4
  Delay2Cycle/1(y) -> Mux/3
  Delay4Cycle/1(y) -> Mux/5
  Bus to Vector/1 -> y/1
  u/1 -> Delay1Cycle/1(u), Delay2Cycle/1(u), Delay3Cycle/1(u), Delay4Cycle/1(u), Mux/1

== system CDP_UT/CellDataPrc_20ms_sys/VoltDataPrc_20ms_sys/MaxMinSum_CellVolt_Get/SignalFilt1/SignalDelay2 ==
  u : Inport
  Bus to Vector : BusToVector
  Delay1Cycle : Subsystem
  Delay2Cycle : Subsystem
  Delay3Cycle : Subsystem
  Delay4Cycle : Subsystem
  Mux : Mux  Inputs=5
  y : Outport
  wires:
  u/1 -> Mux/1, Delay4Cycle/1(u), Delay3Cycle/1(u), Delay2Cycle/1(u), Delay1Cycle/1(u)
  Bus to Vector/1 -> y/1
  Delay4Cycle/1(y) -> Mux/5
  Delay2Cycle/1(y) -> Mux/3
  Delay3Cycle/1(y) -> Mux/4
  Delay1Cycle/1(y) -> Mux/2
  Mux/1 -> Bus to Vector/1

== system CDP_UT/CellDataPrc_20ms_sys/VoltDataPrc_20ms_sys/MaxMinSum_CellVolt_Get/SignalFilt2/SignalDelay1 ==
  u : Inport
  Bus to Vector : BusToVector
  Delay1Cycle : Subsystem
  Delay2Cycle : Subsystem
  Delay3Cycle : Subsystem
  Delay4Cycle : Subsystem
  Mux : Mux  Inputs=5
  y : Outport
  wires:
  Mux/1 -> Bus to Vector/1
  Delay1Cycle/1(y) -> Mux/2
  Delay3Cycle/1(y) -> Mux/4
  Delay2Cycle/1(y) -> Mux/3
  Delay4Cycle/1(y) -> Mux/5
  Bus to Vector/1 -> y/1
  u/1 -> Delay1Cycle/1(u), Delay2Cycle/1(u), Delay3Cycle/1(u), Delay4Cycle/1(u), Mux/1

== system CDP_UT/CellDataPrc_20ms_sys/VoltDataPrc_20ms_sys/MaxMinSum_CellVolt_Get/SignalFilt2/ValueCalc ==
  Output_Value : Inport
  Output_index : Inport  Port=2
  CcCDP_CellVoltFilConfig_numb : Inport  Port=3
  Constant2 : Constant  Value=CDP_CONST1_NUMB
  Constant4 : Constant  Value=CDP_CONST2_NUMB
  Constant6 : Constant  Value=CDP_CONST1_NUMB
  Constant7 : Constant  Value=CDP_CONST2_NUMB
  Product1 : Product  Inputs=*/  OutDataTypeStr=Inherit: Inherit via back propagation
  Product2 : Product  Inputs=*/  OutDataTypeStr=Inherit: Inherit via back propagation
  Selector : Selector  InputPortWidth=5  IndexOptions=Index vector (port)  Indices=[1 3]  OutputSizes=1
  Selector1 : Selector  InputPortWidth=5  IndexOptions=Index vector (port)  Indices=[1 3]  OutputSizes=1
  Sum : Sum  OutDataTypeStr=Inherit: Inherit via back propagation  RndMeth=Zero
  Sum1 : Sum  OutDataTypeStr=Inherit: Inherit via back propagation  RndMeth=Zero
  Output_Value1 : Outport
  Output_index1 : Outport  Port=2
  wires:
  CcCDP_CellVoltFilConfig_numb/1 -> Sum1/1, Sum/1
  Product2/1 -> Selector1/2
  Product1/1 -> Selector/2
  Constant4/1 -> Product1/2
  Sum/1 -> Product1/1
  Output_index/1 -> Selector1/1
  Constant6/1 -> Sum1/2
  Output_Value/1 -> Selector/1
  Constant2/1 -> Sum/2
  Constant7/1 -> Product2/2
  Sum1/1 -> Product2/1
  Selector/1 -> Output_Value1/1
  Selector1/1 -> Output_index1/1

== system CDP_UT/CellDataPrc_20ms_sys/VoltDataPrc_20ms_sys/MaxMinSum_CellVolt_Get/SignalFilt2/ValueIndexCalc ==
  Output_index1 : Inport
  Input_Numb : Inport  Port=2
  InputValueVld : Inport  Port=3
  InputValueUpdate : Inport  Port=4
  Comparison4 : RelationalOperator  Operator===  OutDataTypeStr=boolean
  Constant1 : Constant  Value=CDP_CONST0_NUMB
  EdgeBi : AIWAYS_Powertrain_BMS_lib/Logical Operators/EdgeBi
  InputValueCalc1 : Stateflow chart  TreatAsAtomicUnit=on
  Logical : Logic  OutDataTypeStr=boolean
  Selector2 : Selector  IndexMode=Zero-based  InputPortWidth=5  IndexOptions=Index vector (port)  Indices=[1 3]  OutputSizes=1
  Unit Delay1 : UnitDelay  SampleTime=-1  StateName=StateName
  Output_Numb : Outport
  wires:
  Selector2/1 -> Output_Numb/1
  EdgeBi/1 -> InputValueCalc1/2(Rige)
  Input_Numb/1 -> InputValueCalc1/1(Input_Value)
  Unit Delay1/1 -> InputValueCalc1/3(Old_Value)
  InputValueCalc1/1(Output_Value) -> Unit Delay1/1, Selector2/1
  Output_index1/1 -> Selector2/2
  InputValueVld/1 -> Logical/1
  Constant1/1 -> Comparison4/2
  InputValueUpdate/1 -> Comparison4/1
  Comparison4/1 -> Logical/2
  Logical/1 -> EdgeBi/1

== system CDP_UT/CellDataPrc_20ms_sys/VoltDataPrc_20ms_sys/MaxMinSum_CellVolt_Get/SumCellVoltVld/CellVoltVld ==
  LaCDP_CellVoltVld_flg : Inport
  CcCDP_CellVoltConfig_numb : Inport  Port=2
  CellVolt : ForIterator  ResetStates=reset  IterationSource=external  IterationVariableDataType=int16
  Comparison1 : RelationalOperator  OutDataTypeStr=boolean
  Constant4 : Constant  Value=CcCDP_CellVoltUpdateThrd_numb
  Data Type Conversion : DataTypeConversion
  Logical Operator : Logic  Operator=OR  AllPortsSameDT=off  OutDataTypeStr=boolean
  Logical Operator1 : Logic  AllPortsSameDT=off  OutDataTypeStr=boolean
  Selector : Selector  IndexOptions=Index vector (port)  Indices=[1 3]  OutputSizes=1
  Sum : Sum  OutDataTypeStr=Inherit: Inherit via back propagation  RndMeth=Zero
  Unit Delay : UnitDelay  InitialCondition=ASWTYPE_TRUE  SampleTime=-1  StateName=StateName
  Unit Delay1 : UnitDelay  SampleTime=-1  StateName=StateName
  Unit Delay2 : UnitDelay  SampleTime=-1  StateName=StateName
  LbCDP_AnyCellVoltVld_flg : Outport
  LbCDP_SumCellVoltVld_flg : Outport  Port=2
  LbCDP_CellVoltUpdateVld_flg : Outport  Port=3
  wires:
  Selector/1 -> Logical Operator1/1, Logical Operator/1, Data Type Conversion/1
  CellVolt/1 -> Selector/2
  CcCDP_CellVoltConfig_numb/1 -> CellVolt/1
  Logical Operator/1 -> Unit Delay1/1, LbCDP_AnyCellVoltVld_flg/1  "LbCDP_AnyCellVoltVld_flg"
  LaCDP_CellVoltVld_flg/1 -> Selector/1
  Logical Operator1/1 -> Unit Delay/1, LbCDP_SumCellVoltVld_flg/1  "LbCDP_SumCellVoltVld_flg"
  Unit Delay/1 -> Logical Operator1/2
  Unit Delay1/1 -> Logical Operator/2
  Data Type Conversion/1 -> Sum/2
  Sum/1 -> Comparison1/1, Unit Delay2/1
  Unit Delay2/1 -> Sum/1
  Constant4/1 -> Comparison1/2
  Comparison1/1 -> LbCDP_CellVoltUpdateVld_flg/1  "LbCDP_CellVoltUpdateVld_flg"

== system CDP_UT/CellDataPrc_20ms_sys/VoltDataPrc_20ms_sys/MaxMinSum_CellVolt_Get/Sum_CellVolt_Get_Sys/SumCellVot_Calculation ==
  LcCDP_SumCellVolt_mV : Inport
  Constant : Constant  Value=CDP_MV2V_NUMB
  Constant1 : Constant  Value=CcCDP_CellVoltConfig_numb
  Data Type Conversion : DataTypeConversion
  Divide1 : Product  Inputs=*/  OutDataTypeStr=single
  Divide2 : Product  Inputs=/*  OutDataTypeStr=single
  OverWrite1 : AIWAYS_Powertrain_BMS_lib/Signals/OverWrite  OverWrite_Value=CcCDP_AvgCellVoltOvr_mV  OverWrite_flag=CbCDP_AvgCellVoltOvrSwt_flg
  OverWrite2 : AIWAYS_Powertrain_BMS_lib/Signals/OverWrite  OverWrite_Value=CcCDP_SumCellVoltOvr_V  OverWrite_flag=CbCDP_SumCellVoltOvrSwt_flg
  GcCDP_SumCellVolt_V : Outport
  GcCDP_AvgCellVolt_mV : Outport  Port=2
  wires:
  Divide2/1 -> OverWrite2/1
  Constant/1 -> Divide2/1
  OverWrite2/1 -> GcCDP_SumCellVolt_V/1  "GcCDP_SumCellVolt_V"
  LcCDP_SumCellVolt_mV/1 -> Divide1/1, Divide2/2
  Constant1/1 -> Divide1/2
  Divide1/1 -> Data Type Conversion/1
  Data Type Conversion/1 -> OverWrite1/1
  OverWrite1/1 -> GcCDP_AvgCellVolt_mV/1  "GcCDP_AvgCellVolt_mV"

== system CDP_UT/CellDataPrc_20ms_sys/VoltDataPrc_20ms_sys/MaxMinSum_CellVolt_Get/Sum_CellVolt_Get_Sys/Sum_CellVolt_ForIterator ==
  CcCDP_CellVoltConfig_numb : Inport
  LaCDP_CellVolt_mV : Inport  Port=2
  Add : Sum  OutDataTypeStr=Inherit: Inherit via back propagation
  MaxCellVoltNumbIterator : ForIterator  ResetStates=reset  IterationSource=external  IterationVariableDataType=int16
  Selector : Selector  IndexOptions=Index vector (port)  Indices=[1 3]  OutputSizes=1
  Unit Delay : UnitDelay  SampleTime=-1  StateName=StateName
  LcCDP_SumCellVolt_mV : Outport
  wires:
  Selector/1 -> Add/2  "LcCDP_IniOutputSumCellVolt_mV"
  MaxCellVoltNumbIterator/1 -> Selector/2
  LaCDP_CellVolt_mV/1 -> Selector/1
  CcCDP_CellVoltConfig_numb/1 -> MaxCellVoltNumbIterator/1
  Add/1 -> Unit Delay/1, LcCDP_SumCellVolt_mV/1  "LcCDP_SumCellVolt_mV"
  Unit Delay/1 -> Add/1

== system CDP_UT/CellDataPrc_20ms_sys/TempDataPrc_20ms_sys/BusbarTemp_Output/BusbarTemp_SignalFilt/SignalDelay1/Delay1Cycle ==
  u : Inport
  Constant2 : Constant  Value=ASWTYPE_FALSE
  Switch : Switch  Criteria=u2 ~= 0  Threshold=1  RndMeth=Zero
  Unit Delay1 : UnitDelay  SampleTime=-1  StateName=StateName
  Unit Delay21 : UnitDelay  InitialCondition=1  SampleTime=-1  StateName=StateName
  y : Outport
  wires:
  Switch/1 -> y/1
  u/1 -> Switch/1, Unit Delay1/1
  Unit Delay1/1 -> Switch/3
  Unit Delay21/1 -> Switch/2
  Constant2/1 -> Unit Delay21/1

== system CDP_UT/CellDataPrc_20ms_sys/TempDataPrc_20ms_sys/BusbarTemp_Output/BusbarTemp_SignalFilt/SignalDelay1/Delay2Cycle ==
  u : Inport
  Constant2 : Constant  Value=ASWTYPE_FALSE
  Switch : Switch  Criteria=u2 ~= 0  Threshold=1  RndMeth=Zero
  Unit Delay1 : UnitDelay  SampleTime=-1  StateName=StateName
  Unit Delay2 : UnitDelay  InitialCondition=1  SampleTime=-1  StateName=StateName
  Unit Delay21 : UnitDelay  InitialCondition=1  SampleTime=-1  StateName=StateName
  Unit Delay3 : UnitDelay  SampleTime=-1  StateName=StateName
  y : Outport
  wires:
  Unit Delay3/1 -> Switch/3
  Unit Delay2/1 -> Switch/2
  Constant2/1 -> Unit Delay21/1
  Unit Delay21/1 -> Unit Delay2/1
  Unit Delay1/1 -> Unit Delay3/1
  u/1 -> Unit Delay1/1, Switch/1
  Switch/1 -> y/1

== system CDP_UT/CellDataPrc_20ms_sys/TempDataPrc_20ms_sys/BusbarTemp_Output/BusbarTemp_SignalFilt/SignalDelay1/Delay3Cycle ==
  u : Inport
  Constant2 : Constant  Value=ASWTYPE_FALSE
  Switch : Switch  Criteria=u2 ~= 0  Threshold=1  RndMeth=Zero
  Unit Delay1 : UnitDelay  SampleTime=-1  StateName=StateName
  Unit Delay2 : UnitDelay  InitialCondition=1  SampleTime=-1  StateName=StateName
  Unit Delay21 : UnitDelay  InitialCondition=1  SampleTime=-1  StateName=StateName
  Unit Delay3 : UnitDelay  SampleTime=-1  StateName=StateName
  Unit Delay4 : UnitDelay  InitialCondition=1  SampleTime=-1  StateName=StateName
  Unit Delay5 : UnitDelay  SampleTime=-1  StateName=StateName
  y : Outport
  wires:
  Unit Delay5/1 -> Switch/3
  Unit Delay4/1 -> Switch/2
  Unit Delay3/1 -> Unit Delay5/1
  Unit Delay2/1 -> Unit Delay4/1
  Constant2/1 -> Unit Delay21/1
  Unit Delay21/1 -> Unit Delay2/1
  Unit Delay1/1 -> Unit Delay3/1
  u/1 -> Unit Delay1/1, Switch/1
  Switch/1 -> y/1

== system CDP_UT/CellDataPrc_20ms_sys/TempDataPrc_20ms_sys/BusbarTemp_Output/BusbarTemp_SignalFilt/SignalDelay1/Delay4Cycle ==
  u : Inport
  Constant2 : Constant  Value=ASWTYPE_FALSE
  Switch : Switch  Criteria=u2 ~= 0  Threshold=1  RndMeth=Zero
  Unit Delay{1,3,5,7} (4 alike) : UnitDelay  SampleTime=-1  StateName=StateName
  Unit Delay{2,4,6,21} (4 alike) : UnitDelay  InitialCondition=1  SampleTime=-1  StateName=StateName
  y : Outport
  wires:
  Unit Delay7/1 -> Switch/3
  Unit Delay6/1 -> Switch/2
  Unit Delay5/1 -> Unit Delay7/1
  Unit Delay4/1 -> Unit Delay6/1
  Unit Delay3/1 -> Unit Delay5/1
  Unit Delay2/1 -> Unit Delay4/1
  Constant2/1 -> Unit Delay21/1
  Unit Delay21/1 -> Unit Delay2/1
  Unit Delay1/1 -> Unit Delay3/1
  u/1 -> Unit Delay1/1, Switch/1
  Switch/1 -> y/1

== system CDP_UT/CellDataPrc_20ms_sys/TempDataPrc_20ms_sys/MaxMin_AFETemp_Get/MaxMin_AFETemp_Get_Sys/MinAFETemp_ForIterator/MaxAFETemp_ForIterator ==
  LcCDP_IniOutputAFETemp_C : Inport
  LcCDP_IniOutputAFETempNumb_numb : Inport  Port=2
  LbCDP_IniOutputAFETempVld_flg : Inport  Port=3
  Constant3 : Constant  Value=CcCDP_MaxAFETempIniVal_C
  Logical Operator : Logic  AllPortsSameDT=off  OutDataTypeStr=boolean
  Relational Operator1 : RelationalOperator  Operator=<=  OutDataTypeStr=boolean
  Switch2 : Switch  Criteria=u2 ~= 0
  Switch3 : Switch  Criteria=u2 ~= 0
  Unit Delay External IC : AIWAYS_Powertrain_BMS_lib/Delay Blocks/Unit Delay External IC
  Unit Delay External IC2 : AIWAYS_Powertrain_BMS_lib/Delay Blocks/Unit Delay External IC
  Unit Delay3 : UnitDelay  SampleTime=-1  StateName=StateName
  LcCDP_MaxAFETempNumb_numb : Outport
  LcCDP_MaxAFETemp_C : Outport  Port=2
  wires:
  LbCDP_IniOutputAFETempVld_flg/1 -> Logical Operator/1
  [LbCDP_AFETempMaxSelction_flg] -> Logical Operator/2
  Switch2/1 -> Unit Delay External IC2/1, LcCDP_MaxAFETemp_C/1, Unit Delay External IC/1  "LcCDP_MaxAFETemp_C"
  Unit Delay External IC/1 -> Relational Operator1/1
  Relational Operator1/1 -> [LbCDP_AFETempMaxSelction_flg]  "LbCDP_AFETempMaxSelction_flg"
  LcCDP_IniOutputAFETempNumb_numb/1 -> Switch3/1
  LcCDP_IniOutputAFETemp_C/1 -> Switch2/1, Relational Operator1/2, Unit Delay External IC/2
  Unit Delay External IC2/1 -> Switch2/3
  Logical Operator/1 -> Switch2/2, Switch3/2
  Unit Delay3/1 -> Switch3/3
  Switch3/1 -> Unit Delay3/1, LcCDP_MaxAFETempNumb_numb/1  "LcCDP_MaxAFETempNumb_numb"
  Constant3/1 -> Unit Delay External IC2/2

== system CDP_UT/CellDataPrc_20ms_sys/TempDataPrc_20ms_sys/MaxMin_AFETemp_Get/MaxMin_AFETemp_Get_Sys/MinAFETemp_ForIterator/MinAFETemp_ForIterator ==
  LcCDP_IniOutputAFETemp_C : Inport
  LcCDP_IniOutputAFETempNumb_numb : Inport  Port=2
  LbCDP_IniOutputAFETempVld_flg : Inport  Port=3
  Constant3 : Constant  Value=CcCDP_MinAFETempIniVal_C
  Logical Operator : Logic  AllPortsSameDT=off  OutDataTypeStr=boolean
  Relational Operator3 : RelationalOperator  OutDataTypeStr=boolean
  Switch : Switch  Criteria=u2 ~= 0
  Switch1 : Switch  Criteria=u2 ~= 0
  Unit Delay External IC1 : AIWAYS_Powertrain_BMS_lib/Delay Blocks/Unit Delay External IC
  Unit Delay External IC2 : AIWAYS_Powertrain_BMS_lib/Delay Blocks/Unit Delay External IC
  Unit Delay1 : UnitDelay  SampleTime=-1  StateName=StateName
  LcCDP_MinAFETemp_C : Outport
  LcCDP_MinAFETempNumb_numb : Outport  Port=2
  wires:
  [LbCDP_AFETempMinSelction_flg] -> Logical Operator/2
  LbCDP_IniOutputAFETempVld_flg/1 -> Logical Operator/1
  Unit Delay External IC1/1 -> Relational Operator3/1
  Switch/1 -> Unit Delay External IC2/1, LcCDP_MinAFETemp_C/1, Unit Delay External IC1/1  "LcCDP_MinAFETemp_C"
  LcCDP_IniOutputAFETemp_C/1 -> Switch/1, Relational Operator3/2, Unit Delay External IC1/2
  Logical Operator/1 -> Switch1/2, Switch/2
  Unit Delay External IC2/1 -> Switch/3
  Relational Operator3/1 -> [LbCDP_AFETempMinSelction_flg]  "LbCDP_AFETempMinSelction_flg"
  Unit Delay1/1 -> Switch1/3
  LcCDP_IniOutputAFETempNumb_numb/1 -> Switch1/1
  Switch1/1 -> Unit Delay1/1, LcCDP_MinAFETempNumb_numb/1  "LcCDP_MinAFETempNumb_numb"
  Constant3/1 -> Unit Delay External IC2/2
